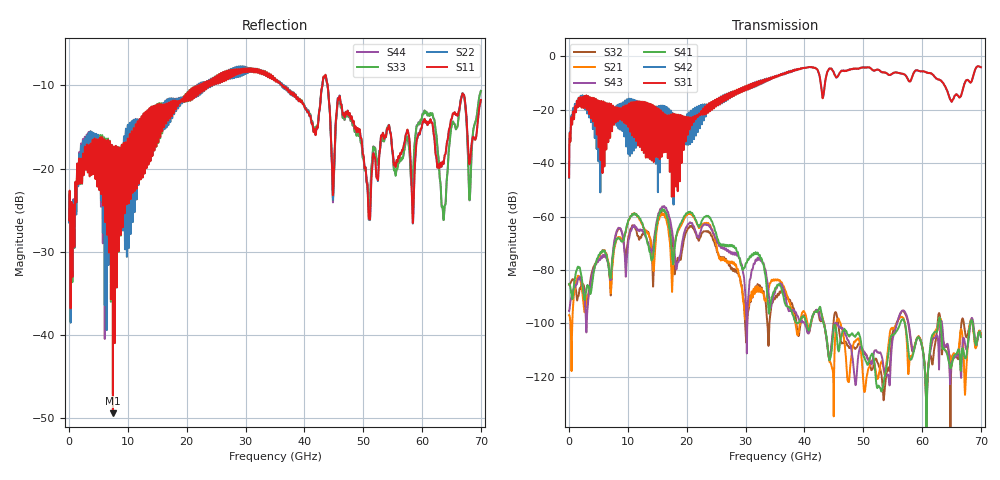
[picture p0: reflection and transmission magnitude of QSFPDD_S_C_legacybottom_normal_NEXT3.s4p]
! AWR Design Environment (8415) Thu Dec 20 15:00:38 2018
! Document = 'CHANNEL TEST'
! nPorts: 4, nXvals: 7001
# HZ S DB R 50
!Freq DBS11 AngS11 DBS12 AngS12 DBS13 AngS13 DBS14 AngS14
!	DBS21 AngS21 DBS22 AngS22 DBS23 AngS23 DBS24 AngS24
!	DBS31 AngS31 DBS32 AngS32 DBS33 AngS33 DBS34 AngS34
!	DBS41 AngS41 DBS42 AngS42 DBS43 AngS43 DBS44 AngS44
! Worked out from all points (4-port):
!   7000 points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, 10 MHz to 70 GHz, reference 50 ohm
!   strongest paths, dB at 10 MHz, 17.51 GHz, 35.01 GHz, 52.51 GHz, 70 GHz:
!     S31: -45.3, -28.7, -7.5, -5.0, -4.0
!     S42: -45.5, -23.8, -7.5, -5.0, -4.0
!     S41: -85.2, -74.1, -87.0, -123.6, -105.1
!     S43: -95.4, -65.2, -88.3, -110.8, -105.0
!     S21: -96.9, -88.2, -83.8, -120.6, -104.1
!     S32: -85.5, -70.0, -90.7, -115.0, -104.1
!   lowest |S11| = -49.4 dB at 7.45 GHz (marker M1), VSWR 1.01, Z = 50.3 + j0.0931 ohm
!   |S11| at or under -10 dB: start of sweep to 22.1 GHz; 36.25 GHz to 43.06 GHz (6.813 GHz wide, 17.2 % of centre); 43.96 GHz to end of sweep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
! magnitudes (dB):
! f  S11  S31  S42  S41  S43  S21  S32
! 10 MHz  -26.2  -45.3  -45.5  -85.2  -95.4  -96.9  -85.5
! 1.65 GHz  -19.7  -15.5  -15.4  -79.1  -83.3  -82.6  -89.2
! 7.45 GHz  -49.4  -18.5  -23.4  -74.6  -73.4  -76.5  -75.1
! 16.1 GHz  -14.0  -33.5  -35.6  -57.5  -56.2  -59.1  -57.6
! 18.37 GHz  -12.0  -23.4  -28.6  -66.0  -78.2  -66.4  -76.5
! 20.62 GHz  -11.8  -23.4  -26.8  -58.2  -62.2  -58.8  -63.5
! 70 GHz  -11.8  -4.0  -4.0  -105.1  -105.0  -104.1  -104.1
